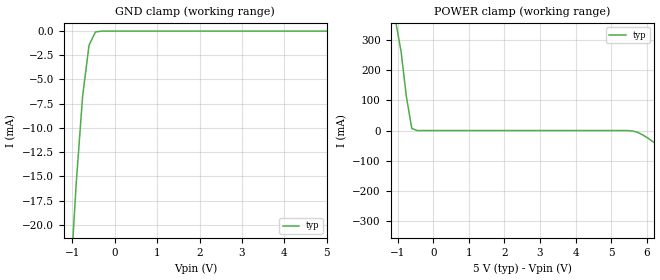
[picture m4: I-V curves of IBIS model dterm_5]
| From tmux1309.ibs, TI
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| dterm_5
[Model]   dterm_5
Model_type   Terminator
|   typ   min   max
C_comp   6.362683e-12   NA   NA
[Voltage Range]   5   NA   NA
[Temperature Range]   27   NA   NA
[Power Clamp Reference]   5   NA   NA
[GND Clamp Reference]   0   NA   NA
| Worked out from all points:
|   GND clamp passes 1 mA (typ) near -0.56 V on its own axis
|   POWER clamp passes 1 mA (typ) near -0.48 V on its own axis
[GND Clamp]
|   Voltage   I(typ)   I(min)   I(max)
-10V      -75.72kA   NA         NA
-1.061V   -27.05mA   NA         NA
-909.1mV  -15.8mA    NA         NA
-757.6mV  -6.756mA   NA         NA
-606.1mV  -1.459mA   NA         NA
-454.5mV  -90.83uA   NA         NA
-303mV    -1.847uA   NA         NA
5V        1.306nA    NA         NA
[POWER Clamp]
|   Voltage   I(typ)   I(min)   I(max)
-5V       1.615A     NA         NA
-1.061V   362.3mA    NA         NA
-909.1mV  263mA      NA         NA
-757.6mV  111.9mA    NA         NA
-606.1mV  6.885mA    NA         NA
-454.6mV  4.888uA    NA         NA
5.606V    -1.459mA   NA         NA
5.909V    -15.8mA    NA         NA
6.364V    -53.24mA   NA         NA
7.879V    -211.1mA   NA         NA
8.03V     -447.2mA   NA         NA
10V       -20.06kA   NA         NA
